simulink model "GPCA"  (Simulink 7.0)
settings: Solver=ode45  StartTime=0.0  StopTime=inf  RelTol=1e-3
PreLoadFcn:
  | GPCA_Bus_Def
InitFcn:
  | script
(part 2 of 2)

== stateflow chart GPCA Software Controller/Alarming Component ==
  state AlarmingMachine
    state WRN [parallel]
      state HumidityCheck
      state BatteryChargingCheck
      state LowBatteryCheck
      state LoggingCheck
      state InfusionPausedDurationCheck
      state EndState
      state WNStart
        en: WnCond = 0;
      state LowReservoirCheck
      state VoltageCheck
      state FlowRateStabilityCheck
      state HoldOn
      state PumpTempCheck
      state EnvTempCheck
      state APErrCheck
      (junction 797) -> (junction 796)
      BatteryChargingCheck -> VoltageCheck : [hardwareSenData.isBatteryUnableToCharge == 0]{clearWarning(21);}
      (junction 798) -> (junction 797)
      LowBatteryCheck -> BatteryChargingCheck : [hardwareSenData.isBatteryLow ==0]{clearWarning(20);}
      LoggingCheck -> LowBatteryCheck : [hardwareSenData.isLoggingFailed == 0]{clearWarning(19);}
      (junction 813) -> LowReservoirCheck : {WnCond := 16; send(E_WarningAlarm, Controller);}
      LowReservoirCheck -> (junction 814) : [infuSenData.isReservoirLow > 0 && infusionInProgress > 0 ]
      (junction 818) -> VoltageCheck : {WnCond := 21; send(E_WarningAlarm, Controller);}
      LowReservoirCheck -> (junction 791) : E_ResetThree
      InfusionPausedDurationCheck -> (junction 792) : E_ResetThree
      LowReservoirCheck -> InfusionPausedDurationCheck : [infuSenData.isReservoirLow == 0 || infusionInProgress == 0 ]{clearWarning(17);}
      LoggingCheck -> (junction 793) : E_ResetThree
      LowBatteryCheck -> (junction 795) : E_ResetThree
      BatteryChargingCheck -> (junction 796) : E_ResetThree
      EndState -> WNStart : E_Clock{send(E_DoneThree, Controller);}
      (junction 823) -> (junction 821)
      VoltageCheck -> (junction 758) : [hardwareSenData.isSupplyVoltageOutOfRange > 0]
      (default) -> WNStart
      WNStart -> HoldOn : E_ResetThree
      HoldOn -> FlowRateStabilityCheck : E_Clock{WnCond := 0;}
      (junction 819) -> EnvTempCheck : {WnCond := 23; send(E_WarningAlarm, Controller);}
      PumpTempCheck -> (junction 819) : [hardwareSenData.isPumpOverheated > 0]
      (junction 816) -> LowBatteryCheck : {WnCond := 19; send(E_WarningAlarm, Controller);}
      VoltageCheck -> (junction 797) : E_ResetThree
      PumpTempCheck -> (junction 798) : E_ResetThree
      (junction 814) -> InfusionPausedDurationCheck : {WnCond := 17; send(E_WarningAlarm, Controller);}
      InfusionPausedDurationCheck -> LoggingCheck : [infuSenData.isInfusionPausedLong == 0 || infusionInProgress == 0 || infusionPaused == 0]{clearWarning(18);}
      (junction 758) -> PumpTempCheck : {WnCond := 22; send(E_WarningAlarm, Controller);}
      (junction 822) -> APErrCheck : {WnCond := 25; send(E_WarningAlarm, Controller);}
      (junction 781) -> WNStart : E_Clock{send(E_DoneThree, Controller);}
      BatteryChargingCheck -> (junction 818) : [hardwareSenData.isBatteryUnableToCharge > 0]
      (junction 817) -> BatteryChargingCheck : {WnCond := 20; send(E_WarningAlarm, Controller);}
      LowBatteryCheck -> (junction 817) : [hardwareSenData.isBatteryLow > 0]
      FlowRateStabilityCheck -> (junction 794) : E_ResetThree
      FlowRateStabilityCheck -> LowReservoirCheck : [infuSenData.isFlowRateNotStable == 0 || infusionInProgress == 0 || infusionPaused == 0]{clearWarning(16);}
      FlowRateStabilityCheck -> (junction 813) : [infuSenData.isFlowRateNotStable > 0 && infusionInProgress > 0 && infusionPaused == 0]
      (junction 794) -> HoldOn
      (junction 791) -> (junction 794)
      (junction 792) -> (junction 791)
      (junction 793) -> (junction 792)
      (junction 795) -> (junction 793)
      (junction 796) -> (junction 795)
      InfusionPausedDurationCheck -> (junction 815) : [infuSenData.isInfusionPausedLong > 0 && infusionInProgress>0 && infusionPaused == 1]
      (junction 815) -> LoggingCheck : {WnCond := 18; send(E_WarningAlarm, Controller);}
      LoggingCheck -> (junction 816) : [hardwareSenData.isLoggingFailed > 0]
      EnvTempCheck -> (junction 821) : E_ResetThree
      EnvTempCheck -> (junction 820) : [envSenData.isTemperatureOutOfRange > 0]
      (junction 820) -> HumidityCheck : {WnCond := 24; send(E_WarningAlarm, Controller);}
      (junction 821) -> (junction 798)
      HumidityCheck -> (junction 823) : E_ResetThree
      HumidityCheck -> (junction 822) : [envSenData.isHumidityOutOfRange > 0]
      APErrCheck -> (junction 781) : [envSenData.isAirPressureOutOfRange ==0]{clearWarning(26);}
      APErrCheck -> (junction 824) : E_ResetThree
      HumidityCheck -> APErrCheck : [envSenData.isHumidityOutOfRange == 0]{clearWarning(25);}
      (junction 824) -> (junction 823)
      VoltageCheck -> PumpTempCheck : [hardwareSenData.isSupplyVoltageOutOfRange == 0]{clearWarning(22);}
      PumpTempCheck -> EnvTempCheck : [hardwareSenData.isPumpOverheated == 0]{clearWarning(23);}
      EnvTempCheck -> HumidityCheck : [envSenData.isTemperatureOutOfRange == 0]{clearWarning(24);}
      APErrCheck -> (junction 825) : [envSenData.isAirPressureOutOfRange > 0]
      (junction 825) -> EndState : {WnCond := 26; send(E_WarningAlarm, Controller);}
    state Controller [parallel]
      state SinkTWOCheckOne
      state START
        en: initiate();
      state CheckLOne
        en:  initiate();
      state CheckWRN
      state SinkOne
      state SinkTWO
      state CheckLTwo
      CheckWRN -> CheckLOne : E_DoneThree{send(E_ResetOne, LOne);}
      SinkOne -> CheckLOne : E_Restart{send(E_ResetOne, LOne);}
      CheckLOne -> SinkOne : E_LevelOneAlarm{ErrCond:=LOneCond;}
      START -> CheckLOne : E_Restart{send(E_ResetOne, LOne);}
      (default) -> START
      CheckWRN -> CheckWRN : E_WarningAlarm{ErrCond:=WnCond; E_Warning}
      CheckLTwo -> CheckWRN : E_DoneTwo{send(E_ResetThree, WRN);}
      SinkTWOCheckOne -> SinkTWO : E_DoneOne
      CheckLTwo -> SinkTWO : E_LevelTwoAlarm{ErrCond:=LTwoCond;}
      SinkTWO -> SinkTWOCheckOne : [LTwoCond>0]{send(E_ResetOne, LOne);}
      CheckLOne -> CheckLTwo : E_DoneOne{send(E_ResetTwo, LTwo);}
      CheckLTwo -> CheckLOne : E_Restart{send(E_ResetOne, LOne);}
      CheckWRN -> CheckLOne : E_Restart{send(E_ResetOne, LOne);}
      SinkTWO -> CheckLOne : E_Restart|E_AlarmClear{ErrCond := 0; send(E_ResetOne, LOne);}
      SinkTWO -> CheckLOne : E_Clock[LTwoCond==0]{ErrCond := 0; send(E_ResetOne, LOne);}
      SinkTWOCheckOne -> CheckLOne : E_Restart|E_AlarmClear{ErrCond := LOneCond; send(E_ResetOne, LOne);}
      SinkTWOCheckOne -> SinkOne : E_LevelOneAlarm{ErrCond:=LOneCond;}
    state LTwo [parallel]
      state Hold
      state Sink24
        en: LTwoCond = 10;
        send(E_LevelTwoAlarm, Controller);
      state Sink26
        en: LTwoCond=12;
        send(E_LevelTwoAlarm, Controller);
      state RateOverPumpCapacityCheck
      state LowInfusionRateCheck
      state RateLessThanKVOCheck
      state Sink25
        en: LTwoCond = 11;
        send(E_LevelTwoAlarm, Controller);
      state OcculusionCheck
      state Sink23
        en: LTwoCond = 9;
        send(E_LevelTwoAlarm, Controller);
      state HighInfusionRateCheck
      state Normal
        en: LTwoCond =0;
      state DoorOpenCheck
      state Sink22
        en: LTwoCond = 8;
        send(E_LevelTwoAlarm, Controller);
      state ReservoirEmptyCheck
      state Sink21
        en: LTwoCond=7;
        send(E_LevelTwoAlarm, Controller);
      state InfusionPauseDurationCheck
      state Sink27
        en: LTwoCond=13;
        send(E_LevelTwoAlarm, Controller);
      state AirInLineCheck
      state Sink29
        en: LTwoCond=15;
        send(E_LevelTwoAlarm, Controller);
      state Sink28
        en: LTwoCond=14;
        send(E_LevelTwoAlarm, Controller);
      AirInLineCheck -> Sink29 : [infuSenData.isAirInLineDetected > 0 && infusionInProgress > 0]
      InfusionPauseDurationCheck -> AirInLineCheck : [infuSenData.isInfusionPausedTooLong == 0  || infusionInProgress == 0 || infusionPaused == 0]
      InfusionPauseDurationCheck -> Sink28 : [infuSenData.isInfusionPausedTooLong > 0  && infusionInProgress > 0 && infusionPaused == 1]
      Sink29 -> (junction 773) : [infuSenData.isAirInLineDetected == 0 || infusionInProgress == 0]
      Sink29 -> (junction 772) : E_ResetTwo
      Sink28 -> (junction 774) : [infuSenData.isInfusionPausedTooLong == 0  || infusionInProgress == 0 || infusionPaused == 0]
      Sink28 -> (junction 775) : E_ResetTwo
      (junction 760) -> DoorOpenCheck
      (junction 773) -> (junction 774)
      AirInLineCheck -> (junction 761) : E_ResetTwo
      InfusionPauseDurationCheck -> (junction 762) : E_ResetTwo
      RateOverPumpCapacityCheck -> InfusionPauseDurationCheck : [infuSenData.isFlowRateOverPumpCapacity == 0 || infusionInProgress == 0]
      Sink27 -> (junction 776) : [infuSenData.isFlowRateOverPumpCapacity == 0 || infusionInProgress == 0]
      RateOverPumpCapacityCheck -> Sink27 : [infuSenData.isFlowRateOverPumpCapacity > 0 && infusionInProgress > 0 ]
      RateOverPumpCapacityCheck -> (junction 812) : E_ResetTwo
      Sink27 -> (junction 777) : E_ResetTwo
      RateLessThanKVOCheck -> RateOverPumpCapacityCheck : [infuSenData.isInfusionRateLessThanKVO == 0 || infusionInProgress == 0]
      Sink26 -> (junction 779) : E_ResetTwo
      RateLessThanKVOCheck -> (junction 811) : E_ResetTwo
      RateLessThanKVOCheck -> Sink26 : [infuSenData.isInfusionRateLessThanKVO > 0 && infusionInProgress > 0]
      Sink26 -> (junction 778) : [infuSenData.isInfusionRateLessThanKVO == 0 || infusionInProgress == 0]
      LowInfusionRateCheck -> RateLessThanKVOCheck : [infuSenData.isInfusionRateTooLow == 0 || infusionInProgress == 0 || infusionPaused > 0]
      Sink25 -> (junction 780) : [infuSenData.isInfusionRateTooLow == 0 || infusionInProgress == 0 || infusionPaused > 0]
      LowInfusionRateCheck -> (junction 810) : E_ResetTwo
      LowInfusionRateCheck -> Sink25 : [infuSenData.isInfusionRateTooLow > 0 && infusionInProgress > 0 && infusionPaused == 0]
      Sink25 -> (junction 769) : E_ResetTwo
      HighInfusionRateCheck -> LowInfusionRateCheck : [infuSenData.isInfusionRateTooHigh == 0 || infusionInProgress == 0 || infusionPaused > 0]
      HighInfusionRateCheck -> Sink24 : [infuSenData.isInfusionRateTooHigh > 0 && infusionInProgress > 0 && infusionPaused == 0]
      OcculusionCheck -> HighInfusionRateCheck : [infuSenData.isOcclusionDetected == 0 || infusionInProgress == 0]
      OcculusionCheck -> Sink23 : [infuSenData.isOcclusionDetected > 0 && infusionInProgress > 0]
      Sink24 -> (junction 756) : E_ResetTwo
      Sink24 -> (junction 757) : [infuSenData.isInfusionRateTooHigh == 0 || infusionInProgress == 0 || infusionPaused > 0]
      Sink23 -> (junction 770) : [infuSenData.isOcclusionDetected == 0 || infusionInProgress == 0]
      Sink23 -> (junction 771) : E_ResetTwo
      ReservoirEmptyCheck -> OcculusionCheck : [infuSenData.isReservoirEmpty == 0 || infusionInProgress == 0]
      ReservoirEmptyCheck -> Sink22 : [infuSenData.isReservoirEmpty > 0 && infusionInProgress > 0]
      ReservoirEmptyCheck -> (junction 807) : E_ResetTwo
      HighInfusionRateCheck -> (junction 809) : E_ResetTwo
      OcculusionCheck -> (junction 808) : E_ResetTwo
      Sink22 -> (junction 766) : [infuSenData.isReservoirEmpty == 0 || infusionInProgress == 0]
      Sink22 -> (junction 767) : E_ResetTwo
      Sink21 -> (junction 764) : [hardwareSenData.isReservoirDoorOpen == 0 || infusionInProgress == 0]
      Sink21 -> (junction 763) : E_ResetTwo
      DoorOpenCheck -> Sink21 : [hardwareSenData.isReservoirDoorOpen > 0 && infusionInProgress > 0]
      DoorOpenCheck -> ReservoirEmptyCheck : [hardwareSenData.isReservoirDoorOpen == 0 || infusionInProgress == 0]
      DoorOpenCheck -> (junction 806) : E_ResetTwo
      (junction 772) -> (junction 775)
      (junction 757) -> (junction 770)
      Hold -> DoorOpenCheck : E_Clock{LTwoCond=0;}
      (junction 756) -> (junction 771)
      (junction 775) -> (junction 777)
      (default) -> Normal
      Normal -> Hold : E_ResetTwo
      (junction 806) -> Hold
      (junction 808) -> (junction 807)
      (junction 809) -> (junction 808)
      (junction 807) -> (junction 806)
      (junction 812) -> (junction 811)
      (junction 811) -> (junction 810)
      (junction 810) -> (junction 809)
      (junction 774) -> (junction 776)
      (junction 761) -> (junction 762)
      (junction 762) -> (junction 812)
      (junction 780) -> (junction 757)
      (junction 769) -> (junction 756)
      (junction 770) -> (junction 766)
      (junction 771) -> (junction 767)
      (junction 766) -> (junction 764)
      (junction 767) -> (junction 763)
      (junction 768) -> DoorOpenCheck : E_Clock
      (junction 764) -> (junction 768)
      (junction 763) -> (junction 760)
      (junction 785) -> Normal : {send(E_DoneTwo, Controller);}
      AirInLineCheck -> (junction 785) : [infuSenData.isAirInLineDetected == 0 || infusionInProgress == 0]
      (junction 776) -> (junction 778)
      (junction 777) -> (junction 779)
      (junction 778) -> (junction 780)
      (junction 779) -> (junction 769)
    state LOne [parallel]
      state HOLD
      state WatchdogCheck
      state MemoryCheck
      state CPUCheck
      state RTCCheck
      state Normal
      state PumpTempCheck
      state L1Sink
      state BatteryDepletionCheck
      (junction 802) -> (junction 800)
      WatchdogCheck -> L1Sink : [hardwareSenData.isWatchDogInterruptDetected > 0]{LOneCond:=6; send(E_LevelOneAlarm, Controller);}
      PumpTempCheck -> WatchdogCheck : [hardwareSenData.isPumpTooHot == 0]
      Normal -> HOLD : E_ResetOne
      WatchdogCheck -> (junction 805) : [hardwareSenData.isWatchDogInterruptDetected==0]{send(E_DoneOne, Controller);}
      WatchdogCheck -> (junction 786) : E_ResetOne
      (default) -> Normal
      L1Sink -> HOLD : E_ResetOne
      PumpTempCheck -> L1Sink : [hardwareSenData.isPumpTooHot >0]{LOneCond:=5; send(E_LevelOneAlarm, Controller);}
      MemoryCheck -> PumpTempCheck : [hardwareSenData.isMemoryCorrupted == 0]
      MemoryCheck -> L1Sink : [hardwareSenData.isMemoryCorrupted > 0]{LOneCond:=4; send(E_LevelOneAlarm, Controller);}
      CPUCheck -> MemoryCheck : [hardwareSenData.isCPUInError == 0]
      CPUCheck -> L1Sink : [hardwareSenData.isCPUInError > 0]{LOneCond := 3; send(E_LevelOneAlarm, Controller);}
      RTCCheck -> CPUCheck : [hardwareSenData.isRTCInError > 0 == 0]
      RTCCheck -> L1Sink : [hardwareSenData.isRTCInError > 0> 0]{LOneCond:=2; send(E_LevelOneAlarm, Controller);}
      BatteryDepletionCheck -> RTCCheck : [hardwareSenData.isBatteryDepleted == 0]
      BatteryDepletionCheck -> L1Sink : [hardwareSenData.isBatteryDepleted > 0]{LOneCond:=1; send(E_LevelOneAlarm, Controller);}
      MemoryCheck -> (junction 803) : E_ResetOne
      PumpTempCheck -> (junction 804) : E_ResetOne
      CPUCheck -> (junction 802) : E_ResetOne
      RTCCheck -> (junction 800) : E_ResetOne
      BatteryDepletionCheck -> (junction 799) : E_ResetOne
      (junction 799) -> HOLD
      HOLD -> BatteryDepletionCheck : E_Clock{LOneCond=0;}
      (junction 786) -> (junction 804)
      (junction 805) -> Normal : E_Clock
      (junction 804) -> (junction 803)
      (junction 800) -> (junction 799)
      (junction 803) -> (junction 802)
    state CheckReady [parallel]
      state Normal
      state s1
      state Checking
        en: temp := isPumpReady();
      state s2
      s2 -> Normal : E_Restart
      s2 -> s2 : E_Clock{E_NotReady}
      s1 -> Normal : E_Restart
      s1 -> s1 : E_Clock[infusionInProgress == 0]{E_Ready}
      Checking -> Normal : E_Restart
      s2 -> Checking : E_RequestToStart
      s1 -> Normal : E_Clock[infusionInProgress == 1]
      s1 -> Checking : E_RequestToStart
      (default) -> Normal
      Normal -> Checking : E_RequestToStart
      Checking -> s2 : [temp == 0]
      Checking -> s1 : [temp > 0]
    (default) -> Controller
  state x = clearWarning(cond) [function]
    (junction 784) -> (junction 783) : [ErrCond != cond]{x:=0;}
    (junction 784) -> (junction 782) : [ErrCond == cond]{ml.GAlrmMsg = MSG_BLANK; ErrCond := 0;}
    (default) -> (junction 784)
  state x = isPumpReady [function]
    (junction 765) -> (junction 787) : [infuSenData.isReservoirEmpty > 0]{ x := 0;}
    (junction 759) -> (junction 789) : [hardwareSenData.isReservoirDoorOpen > 0] {x := 0;}
    (junction 765) -> (junction 759) : [infuSenData.isReservoirEmpty == 0]
    (default) -> (junction 765)
    (junction 759) -> (junction 788) : [hardwareSenData.isReservoirDoorOpen == 0]
    (junction 788) -> (junction 801) : [infuSenData.isFlowRateOverPumpCapacity > 0]{x := 0;}
    (junction 788) -> (junction 790) : [infuSenData.isFlowRateOverPumpCapacity == 0]{x := 1;}
  state x = initiate [function]
    (default) -> (junction 755) : {LOneCond := 0; LTwoCond := 0; WnCond := 0; ErrCond := 0; x:=0;}
  (default) -> AlarmingMachine

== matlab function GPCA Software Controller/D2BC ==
function y = d_to_b(u)
% This block supports the Embedded MATLAB subset.
% See the help menu for details. 

y = false;

if (u == 0)
    y = false;
else 
     y = true;
end;
